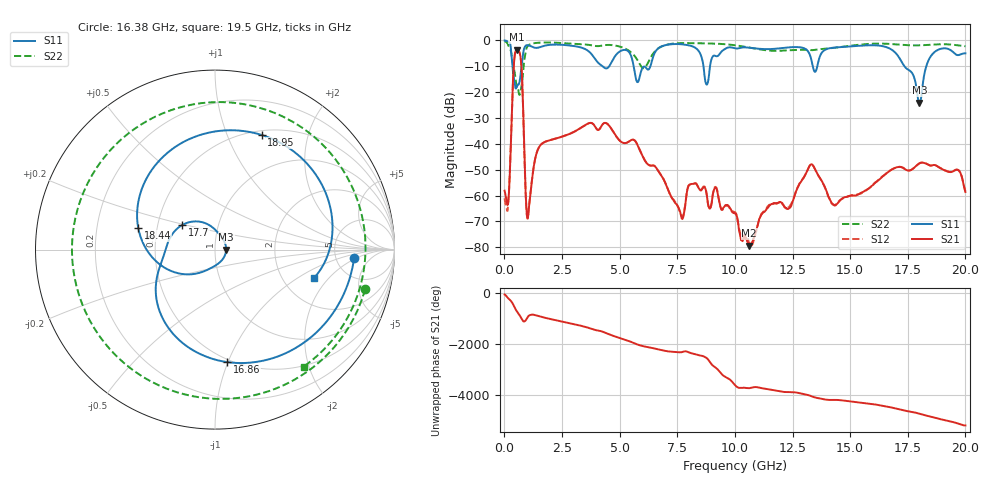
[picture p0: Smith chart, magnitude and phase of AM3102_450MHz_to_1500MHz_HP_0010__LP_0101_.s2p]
!Agilent Technologies,E8364B,MY43040894,A.07.50.67
!Agilent E8364B: A.07.50.67
!Date: Thursday, January 11, 2018 05:24:55
!Correction: S11(Full 2 Port(1,2))
!S21(Full 2 Port(1,2))
!S12(Full 2 Port(1,2))
!S22(Full 2 Port(1,2))
!S2P File: Measurements: S11, S21, S12, S22:
# Hz S  dB  R 50
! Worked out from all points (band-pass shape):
!   1601 points, 10 MHz to 20 GHz, reference 50 ohm
!   highest |S21| = -3.61 dB at 547.2 MHz (marker M1); lowest = -79.3 dB at 10.62 GHz (marker M2)
!   |S21| within 3 dB of the highest: 438.5 MHz to 702.1 MHz (263.6 MHz wide, 46.2 % of centre)
!   lowest |S11| = -24.1 dB at 18 GHz (marker M3), VSWR 1.13, Z = 56.6 + j0.0377 ohm
!   |S11| at or under -10 dB: 349.8 MHz to 744.6 MHz (394.8 MHz wide, 72.1 % of centre); 5.608 GHz to 6.336 GHz (728 MHz wide, 12.2 % of centre); 17.35 GHz to 18.3 GHz (950.4 MHz wide, 5.33 % of centre)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
!   |S22| runs from -21.0 to -0.4 dB; largest |S21 - S12| = 0.0033
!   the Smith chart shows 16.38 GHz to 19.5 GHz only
!   S11 on the Smith chart (normalised r, x): 16.38 GHz: 7.48, -1.83; 16.86 GHz: 0.48, -0.99; 17.7 GHz: 0.67, +0.19; 18.44 GHz: 0.39, +0.12; 18.95 GHz: 0.55, +1.34; 19.5 GHz: 2.99, -1.39
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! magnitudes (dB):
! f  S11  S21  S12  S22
! 10 MHz  -0.1  -58.2  -61.1  -0.4
! 184.9 MHz  -0.6  -60.8  -60.9  -2.4
! 547.2 MHz  -18.0  -3.6  -3.6  -17.8
! 722.1 MHz  -11.7  -8.1  -8.1  -18.8
! 1.022 GHz  -1.9  -68.4  -68.8  -2.1
! 1.534 GHz  -2.7  -40.9  -40.9  -0.9
! 3.346 GHz  -2.8  -33.7  -33.7  -1.5
! 6.682 GHz  -3.0  -50.6  -50.6  -3.1
! 8.781 GHz  -17.1  -59.7  -59.7  -1.2
! 10.01 GHz  -3.1  -67.0  -66.4  -1.9
! 10.62 GHz  -2.8  -79.3  -78.5  -2.8
! 13.34 GHz  -8.4  -47.9  -48.0  -3.8
! 14.32 GHz  -2.8  -63.8  -63.7  -2.9
! 16.38 GHz  -2.2  -52.9  -52.8  -1.3
! 16.68 GHz  -3.0  -50.8  -50.7  -1.4
! 16.86 GHz  -4.0  -49.7  -49.7  -1.5
! 17.7 GHz  -12.8  -49.8  -49.8  -2.0
! 18 GHz  -24.1  -47.6  -47.6  -1.9
! 18.44 GHz  -7.0  -48.3  -48.3  -1.7
! 18.95 GHz  -3.2  -49.6  -49.5  -1.5
! 19.5 GHz  -4.8  -50.5  -50.4  -1.7
! 20 GHz  -5.1  -58.6  -58.3  -2.3
